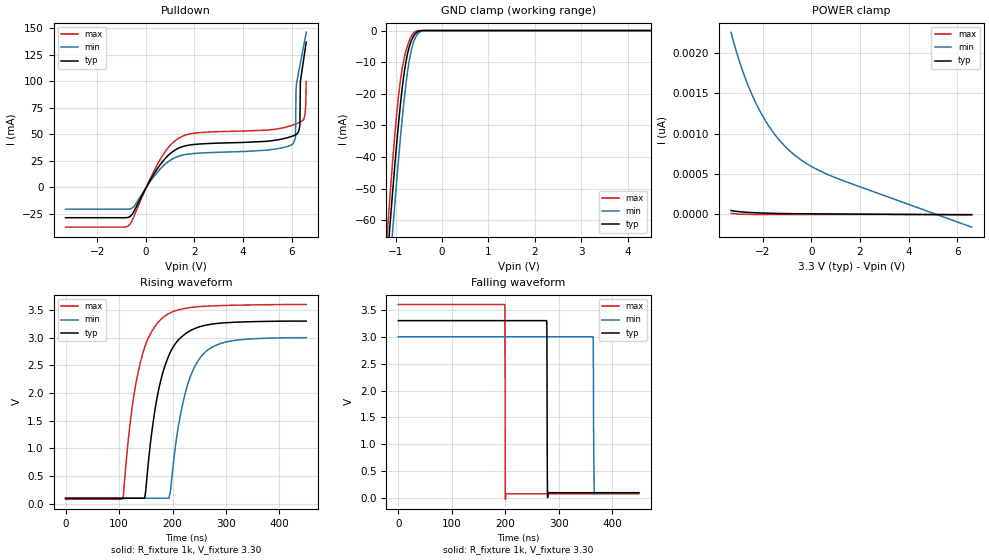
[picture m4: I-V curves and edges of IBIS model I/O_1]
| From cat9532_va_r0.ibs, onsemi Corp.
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|//////////////////////////////////////////////////////////////////////////////
|//////////////////////////////////////////////////////////////////////////////
[Model] I/O_1
Model_type I/O_open_drain
Enable Active-Low
Polarity Non-Inverting
Vinh = 2.31
Vinl = 0.99
Vref = 3.3V
Vmeas = 1.65
Rref = 1k
Cref = 400pF
|  variable   typ   min   max
C_comp   3.275pF   3.275pF   3.275pF
|//////////////////////////////////////////////////////////////////////////////
[Temperature Range]   25   85   -40
|//////////////////////////////////////////////////////////////////////////////
[Voltage Range]   3.30V   3.0V   3.60V
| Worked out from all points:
|   slope of the pulldown table from 0 to 0.495 V, typ, clamps not added: 25.9 ohm
|   GND clamp passes 1 mA (typ) near -0.58 V on its own axis
|   falling waveform, R_fixture 1k, V_fixture 3.30: 20-80 % time 488ps typ, 825ps min, 391ps max; typ from 3.3 V to 0.1 V
|   rising waveform, R_fixture 1k, V_fixture 3.30: 20-80 % time 37.6ns typ, 37.6ns min, 36.9ns max; typ from 0.1 V to 3.3 V
|//////////////////////////////////////////////////////////////////////////////
[Pulldown]
|   Voltage   I(typ)   I(min)   I(max)
-3.3V     -28.5mA    -20.44mA   -37.41mA
-680mV    -27.78mA   -20.36mA   -35.37mA
600mV     21.73mA    17.62mA    26.76mA
1.5V      38.43mA    30.49mA    48.23mA
6.02V     48.31mA    40.56mA    58.69mA
6.16V     49.61mA    48.03mA    59.82mA
6.18V     49.86mA    91.17mA    59.99mA
6.34V     58.78mA    115mA      61.56mA
6.36V     100.1mA    117.4mA    61.78mA
6.54V     127.9mA    139.1mA    67.82mA
6.58V     134.1mA    143.9mA    77.6mA
6.6V      137.1mA    146.3mA    100.1mA
|//////////////////////////////////////////////////////////////////////////////
[GND Clamp]
|   Voltage   I(typ)   I(min)   I(max)
-3.3V     -520.7mA   -505.6mA   -540.5mA
-1.18V    -72.72mA   -85.88mA   -64.53mA
-1.14V    -65.32mA   -78.09mA   -56.32mA
-1.1V     -57.8mA    -70.41mA   -48.38mA
-1.06V    -50.48mA   -62.91mA   -40.83mA
-940mV    -29.95mA   -41.32mA   -21.18mA
-900mV    -23.96mA   -34.65mA   -16.21mA
-820mV    -13.92mA   -22.52mA   -9.086mA
-700mV    -4.888mA   -9.074mA   -3.037mA
-580mV    -1.05mA    -2.429mA   -344.5uA
-340mV    -798.8nA   -12.2uA    -12.72nA
6.6V      14.43pA    982.3pA    494.2fA
|//////////////////////////////////////////////////////////////////////////////
[POWER Clamp]
|   Voltage   I(typ)   I(min)   I(max)
-3.3V     49.24pA    2.259nA    14.12pA
-3.04V    37.28pA    1.979nA    6.226pA
-2.76V    29.33pA    1.727nA    2.158pA
-2.48V    23.9pA     1.514nA    674.8fA
-2.16V    19.64pA    1.31nA     438.2fA
-1.84V    16.41pA    1.14nA     416.8fA
-1.48V    13.26pA    983.8pA    392.8fA
-1.08V    10.97pA    845.1pA    366.1fA
-680mV    9.385pA    735.1pA    339.4fA
40mV      7.996pA    589.7pA    291.4fA
960mV     6.224pA    459.5pA    230fA
6.6V      -4.638pA   -157.2pA   -146.3fA
|//////////////////////////////////////////////////////////////////////////////
|//////////////////////////////////////////////////////////////////////////////
[Ramp]
|  variable   typ   min   max
dV/dt_r   1.920E+00/2.500E-10  1.740E+00/2.500E-10  2.112E+00/2.000E-10
dV/dt_f   1.920E+00/5.000E-10  1.740E+00/8.000E-10  2.112E+00/3.000E-10
R_load = 1k
|//////////////////////////////////////////////////////////////////////////////
[Falling Waveform]
R_fixture = 1k
V_fixture = 3.30
V_fixture_min = 3.0
V_fixture_max = 3.60
C_fixture = 0p
|   time   V(typ)   V(min)   V(max)
0s        3.3V       3V         3.6V
199ns     3.3V       3V         3.599V
199.4ns   3.3V       3V         3.286V
200ns     3.3V       3V         350.5mV
200.3ns   3.3V       3V         -23.13mV
277.4ns   3.3V       3V         80mV
279.1ns   8.536mV    3V         80mV
364.2ns   100mV      3V         80mV
366.7ns   100mV      69.94mV    80mV
450ns     100mV      100mV      80mV
|//////////////////////////////////////////////////////////////////////////////
[Rising Waveform]
R_fixture = 1k
V_fixture = 3.30
V_fixture_min = 3.0
V_fixture_max = 3.60
C_fixture = 0p
|   time   V(typ)   V(min)   V(max)
0s        100mV      100mV      80mV
106ns     100mV      100mV      86.43mV
126ns     100mV      100mV      1.847V
148ns     103.1mV    100mV      2.829V
164ns     1.488V     100mV      3.158V
182ns     2.372V     100mV      3.365V
196ns     2.739V     209.2mV    3.451V
226ns     3.084V     2.077V     3.534V
255ns     3.21V      2.679V     3.565V
450ns     3.3V       3V         3.6V
